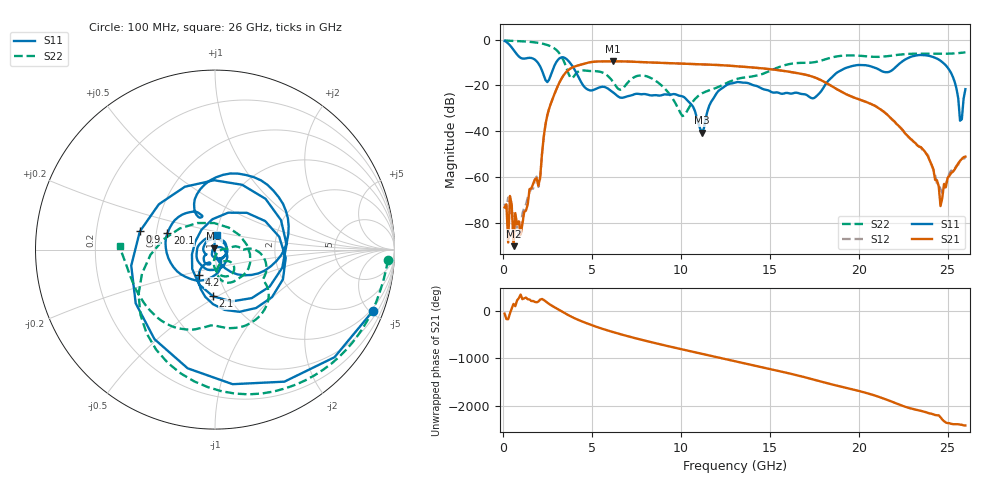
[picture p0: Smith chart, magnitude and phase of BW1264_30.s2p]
!Keysight Technologies,N5245B,MY57181159,A.13.60.06
!Date: Friday, December 18, 2020 23:53:31
!Correction: S11(Full 2 Port(1,2))
!S21(Full 2 Port(1,2))
!S12(Full 2 Port(1,2))
!S22(Full 2 Port(1,2))
!S2P File: Measurements: S11, S21, S12, S22:
# Hz S  dB  R 50
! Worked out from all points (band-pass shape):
!   260 points, 100 MHz to 26 GHz, reference 50 ohm
!   highest |S21| = -9.44 dB at 6.2 GHz (marker M1); lowest = -90.3 dB at 600 MHz (marker M2)
!   |S21| within 3 dB of the highest: 3.835 GHz to 14.5 GHz (10.66 GHz wide, 116 % of centre)
!   lowest |S11| = -40.7 dB at 11.2 GHz (marker M3), VSWR 1.02, Z = 49.5 + j0.783 ohm
!   |S11| at or under -10 dB: 1.963 GHz to 2.99 GHz (1.028 GHz wide, 41.5 % of centre); 3.766 GHz to 22.36 GHz (18.6 GHz wide, 142 % of centre); 24.74 GHz to end of sweep
!   |S22| runs from -33.4 to -0.3 dB; largest |S21 - S12| = 0.00053
!   S11 on the Smith chart (normalised r, x): 100 MHz: 0.83, -5.17; 900 MHz: 0.40, +0.10; 2.1 GHz: 0.86, -0.48; 4.2 GHz: 0.80, -0.23; 20.1 GHz: 0.57, +0.11; 26 GHz: 1.01, +0.17
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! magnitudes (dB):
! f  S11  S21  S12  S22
! 100 MHz  -0.5  -73.3  -71.7  -0.3
! 300 MHz  -1.6  -88.7  -69.0  -0.4
! 400 MHz  -2.4  -68.3  -71.0  -0.4
! 600 MHz  -4.4  -90.3  -75.9  -0.5
! 900 MHz  -7.3  -79.4  -86.4  -0.6
! 2.1 GHz  -11.7  -60.1  -60.6  -1.5
! 2.7 GHz  -15.4  -27.9  -27.9  -2.9
! 4.2 GHz  -15.5  -11.3  -11.3  -14.1
! 4.5 GHz  -19.8  -10.7  -10.6  -13.4
! 6.2 GHz  -23.0  -9.4  -9.4  -18.5
! 8.8 GHz  -24.4  -10.1  -10.1  -19.2
! 10.1 GHz  -24.8  -10.4  -10.5  -33.4
! 11.2 GHz  -40.7  -10.8  -10.8  -23.4
! 13.1 GHz  -18.6  -11.6  -11.6  -17.3
! 17.4 GHz  -25.6  -16.1  -16.1  -9.9
! 20.1 GHz  -11.0  -26.3  -26.3  -7.0
! 21.7 GHz  -14.1  -33.5  -33.5  -7.1
! 23.9 GHz  -6.9  -51.1  -50.5  -6.1
! 24.6 GHz  -9.2  -72.8  -65.3  -6.1
! 25.4 GHz  -18.5  -56.7  -56.4  -6.0
! 25.7 GHz  -35.4  -53.0  -52.6  -5.8
! 26 GHz  -21.6  -51.1  -51.6  -5.5
